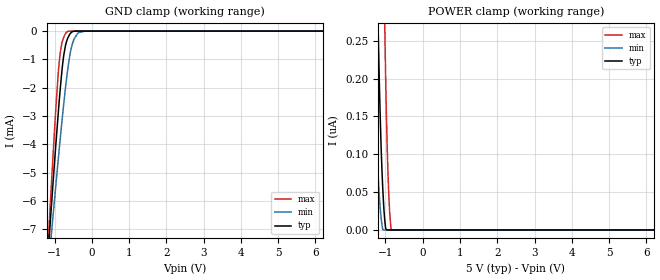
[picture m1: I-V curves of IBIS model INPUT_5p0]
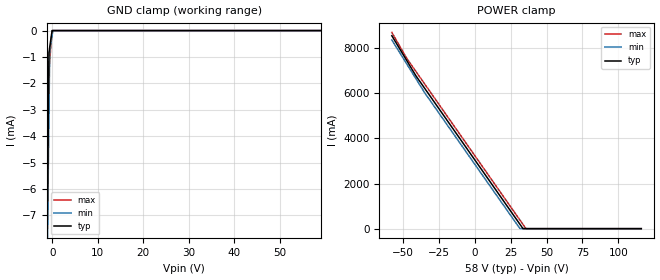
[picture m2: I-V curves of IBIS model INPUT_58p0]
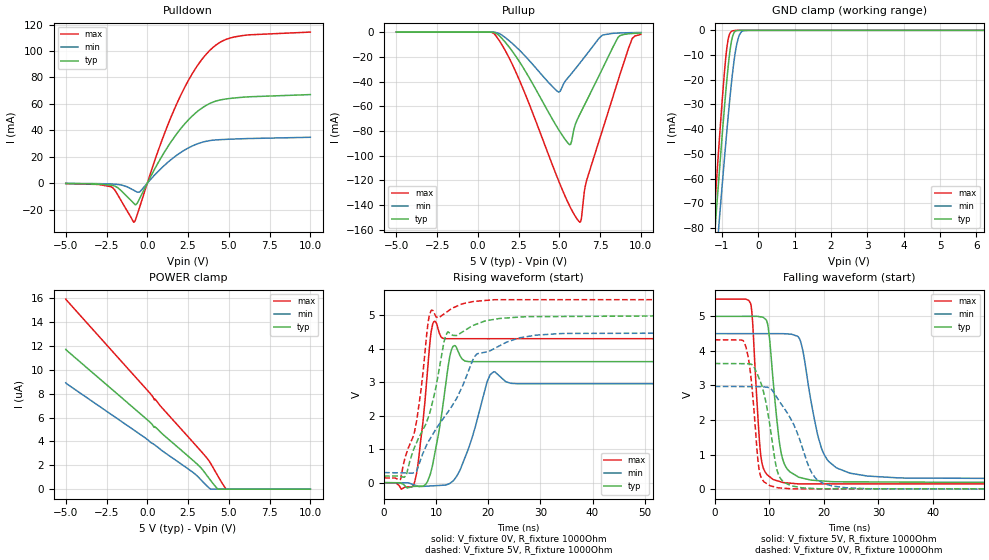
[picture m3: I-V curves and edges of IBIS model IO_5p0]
|Texas Instruments Incorporated
|TPS40170 4.5 V to 60 V, Wide-Input Synchronous PWM Buck Controller
[IBIS Ver]   4.1
[File name]   tps40170.ibs
[Date]   11/27/2018
[File Rev]   1.0
[Source]
| Texas Instruments Incorporated.
| Analog-eLab Design Center, HPA
| 12500 TI Blvd
| Dallas, TX -75243
[Notes]   Revision History:
| Rev 1.0: 11/27/2018
| - Initial version of the model
| - Model generated from simulations in SPECTRE
| - Warnings regarding combined Non-monotonicity of various models
|   have been reviewed and considered minor and can be ignored.
| - C_comp although listed in numerical order of value are
|   obtained from varying PVT conditions. For PVT conditions for
|   each specific value refer the buffer description under
|   respective [Model]. IBIS model user is responsible for using
|   appropriate C_comp to simulate for Signal Integrity.
| - Notes regarding non-monotonicity of various models
|   have been reviewed and considered minor and can be ignored.
| - Model names with a trailing _5 contain the model for 1.8V operation.
|   Model names with a trailing _58 contain the model for 3.3V operation.
|   Model names with a trailing _8 contain the model for 5.0V operation.
[Disclaimer]
| This model is designed as an aid for customers of Texas Instruments.
| TI and its licensors and suppliers make no warranties, either expressed
| or implied, with respect to this  model, including the warranties of
| merchantability or fitness for a particular purpose. The model is
| provided solely on an "as is" basis. The entire risk as to its quality
| and performance is with the customer.
| This model is subject to change without notice. Texas Instruments
| Incorporated is not responsible for updating this model.
[Copyright]
(C) Copyright 2018 Texas Instruments Incorporated.All rights reserved.
|  Component TPS40170RGY 20-pin VQFN - RGY package
|  Part # TPS40170RGY
[Component]   TPS40170RGY
[Manufacturer]  TI
[Package]   |20 VQFN - RGY package
|   typ   min   max
R_pkg   0.05   0.04   0.06
L_pkg   1.0nH   0.8nH   1.2nH
C_pkg   0.2pF   0.16pF   0.24pF
[Pin] signal_name   model_name   R_pin   L_pin   C_pin
1   ENABLE   INPUT   NA   NA   NA
2   SYNC   IO   NA   NA   NA
3   M/S   NC   NA   NA   NA
4   RT   NC   NA   NA   NA
5   SS   NC   NA   NA   NA
6   TRK   NC   NA   NA   NA
7   FB   NC   NA   NA   NA
8   COMP   NC   NA   NA   NA
9   AGND   GND   NA   NA   NA
10   VDD   POWER   NA   NA   NA
11   PGOOD   NC   NA   NA   NA
12   ILIM   NC   NA   NA   NA
13   PGND   GND   NA   NA   NA
14   LDRV   NC   NA   NA   NA
15   VBP   NC   NA   NA   NA
16   SW   NC   NA   NA   NA
17   HDRV   NC   NA   NA   NA
18   BOOT   NC   NA   NA   NA
19   VIN   POWER   NA   NA   NA
20   UVLO   NC   NA   NA   NA
[Model Selector] INPUT
INPUT_5p0   5.0V   digital Input
INPUT_58p0   58.0V  digital Input
[Model Selector] IO
IO_5p0   5.0V  digital I/O
IO_8p0   8.0V  digital I/O
| Models and submodels in the file (4): INPUT_5p0 (Input), INPUT_58p0 (Input), IO_5p0 (I/O), IO_8p0 (I/O)
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|   INPUT_5p0 Model
[Model]   INPUT_5p0
Model_type   Input
Vinl = 0.1
Vinh = 0.6
|   typ   min   max
C_comp   4.463E-13   4.443E-13   4.804E-13
|  Where Nom  PVT is Nominal Process, 5.0V,  27C
|   Fast PVT is Strong Process,  5.5V, -40C
|   Slow PVT is Weak Process,   4.5V, 125C
[Voltage Range]   5   4.5   5.5
|Junction Temperature
[Temperature Range]   27   125   -40
[Power Clamp Reference]   5   4.5   5.5
[GND Clamp Reference]   0   0   0
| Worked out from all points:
|   GND clamp passes 1 mA (typ) near -0.77 V on its own axis
[GND Clamp]
|   Voltage   I(typ)   I(min)   I(max)
-5V       -86.97mA   -70.6mA    -108.1mA
-1.25V    -9.29mA    -9.605mA   -9.357mA
-1.13V    -6.99mA    -7.811mA   -6.43mA
-1.07V    -5.864mA   -6.927mA   -5.009mA
-965mV    -3.955mA   -5.407mA   -2.669mA
-860mV    -2.197mA   -3.939mA   -875.2uA
-755mV    -847.5uA   -2.559mA   -211.6uA
-650mV    -253.7uA   -1.36mA    -12.81uA
-560mV    -56.52uA   -634.1uA   -388.1nA
-470mV    -3.429uA   -258.8uA   -54.84nA
-170mV    -39.22nA   -485.2nA   -50.33nA
10V       0A         0A         0A
[POWER Clamp]
|   Voltage   I(typ)   I(min)   I(max)
-5V       66.16uA    47.89uA    96.51uA
-1.655V   2.175uA    1.129uA    4.477uA
-1.25V    408.6nA    131nA      1.384uA
-1.205V   286.4nA    79.41nA    1.113uA
-1.19V    250.8nA    65.2nA     1.029uA
-1.115V   107.4nA    15.29nA    642.3nA
-1.07V    52.12nA    72.28pA    448.7nA
-1.025V   16.43nA    0A         288.1nA
-935mV    0A         0A         79.11nA
-890mV    0A         0A         25.91nA
-845mV    0A         0A         276.1pA
10V       0A         0A         0A
|   INPUT_58p0 Model
[Model]   INPUT_58p0
Model_type   Input
Vinl = 0.1
Vinh = 0.6
|   typ   min   max
C_comp   4.760E-13   3.805E-13   4.871E-13
|  Where Nom  PVT is Nominal Process, 58V,  27C
|   Fast PVT is Strong Process,  60V, -40C
|   Slow PVT is Weak Process,   56V, 125C
[Voltage Range]   58   56   60
|Junction Temperature
[Temperature Range]   27   125   -40
[Power Clamp Reference]   58   56   60
[GND Clamp Reference]   0   0   0
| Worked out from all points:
|   GND clamp passes 1 mA (typ) near -0.76 V on its own axis
[GND Clamp]
|   Voltage   I(typ)   I(min)   I(max)
-58V      -5.49A     -5.046A    -5.928A
-2.146V   -27.23mA   -23.55mA   -32.3mA
-928mV    -4.137mA   -5.827mA   -1.934mA
-754mV    -838.2uA   -3.295mA   -1.547mA
-580mV    -628.6uA   -762.6uA   -1.16mA
-58mV     -20.47fA   -190.7uA   -51.12fA
116mV     0A         0A         0A
116V      0A         0A         0A
[POWER Clamp]
|   Voltage   I(typ)   I(min)   I(max)
-58V      8.556A     8.365A     8.702A
-47.39V   7.432A     7.282A     7.532A
-40.95V   6.754A     6.626A     6.947A
-34.68V   6.186A     5.99A      6.378A
31.44V    186.8mA    6.365mA    373.9mA
33.52V    5.407mA    346.3uA    185.3mA
35.79V    335uA      268.4uA    503.6uA
116V      0A         0A         0A
|   IO_5p0 Model
[Model]   IO_5p0
Model_type   I/O
Polarity   Non-Inverting
Enable   Active-High
Vinl = 0.8
Vinh = 2
Vmeas = 2.5
Vref = 0
Cref = 2pF
Rref = 100000
|   typ   min   max
C_comp   2.387E-12   1.948E-12   2.498E-12
|  Where Nom  PVT is Nominal Process, 5.0V,  27C
|   Fast PVT is Strong Process,  5.5V, -40C
|   Slow PVT is Weak Process,   4.5V, 125C
[Voltage Range]   5   4.5   5.5
|Junction Temperature
[Temperature Range]   27   125   -40
[Pullup Reference]   5   4.5   5.5
[Pulldown Reference]   -0   0   0
[Power Clamp Reference]   5   4.5   5.5
[GND Clamp Reference]   0   0   0
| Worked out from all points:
|   slope of the pulldown table from 0 to 0.75 V, typ, clamps not added: 43.5 ohm
|   slope of the pullup table from 0 to 0.75 V, typ, clamps not added: 36 kohm
|   GND clamp passes 1 mA (typ) near -0.67 V on its own axis
|   falling waveform, V_fixture 5V, R_fixture 1000Ohm: 20-80 % time 1.82ns typ, 3.13ns min, 1.2ns max; typ from 4.99 V to 0.198 V
|   rising waveform, V_fixture 0V, R_fixture 1000Ohm: 20-80 % time 2.25ns typ, 3.56ns min, 1.65ns max; typ from 0 V to 3.63 V
|   rising waveform, V_fixture 5V, R_fixture 1000Ohm: 20-80 % time 5.18ns typ, 8.8ns min, 3.05ns max; typ from 0.198 V to 4.99 V
|   falling waveform, V_fixture 0V, R_fixture 1000Ohm: 20-80 % time 2.38ns typ, 4.83ns min, 1.43ns max; typ from 3.63 V to 0 V
[Pulldown]
|   Voltage   I(typ)   I(min)   I(max)
-5V       -233.1uA   -135.6uA   -319.7uA
-2.165V   -1.626mA   -658.4uA   -3.098mA
-800mV    -15.63mA   -5.555mA   -29.46mA
-620mV    -15.28mA   -6.757mA   -23.97mA
-455mV    -11.28mA   -6.464mA   -17.64mA
640mV     14.89mA    8.596mA    23.64mA
1.69V     35.41mA    20.08mA    56.84mA
2.74V     50.64mA    28.03mA    82.5mA
3.79V     60.07mA    32.14mA    99.97mA
4.495V    63.05mA    32.96mA    106.9mA
5.47V     64.65mA    33.48mA    111mA
10V       67.05mA    34.74mA    114.4mA
[GND Clamp]
|   Voltage   I(typ)   I(min)   I(max)
-5V       -893.1mA   -848.5mA   -967.2mA
-1.25V    -92.33mA   -109.2mA   -82.83mA
-1.13V    -68.55mA   -87.15mA   -56.65mA
-1.07V    -56.91mA   -76.29mA   -43.93mA
-935mV    -31.84mA   -52.49mA   -17.5mA
-875mV    -21.64mA   -42.35mA   -8.248mA
-800mV    -10.7mA    -30.31mA   -1.899mA
-710mV    -2.577mA   -17.45mA   -244.9uA
-590mV    -85.03uA   -5.428mA   -18.61uA
-515mV    -7.368uA   -1.701mA   -2.317uA
-410mV    -77.06nA   -152uA     0A
10V       0A         0A         0A
[Pullup]
|   Voltage   I(typ)   I(min)   I(max)
-5V       1.348nA    7.768nA    176.2pA
1.045V    -456uA     -166uA     -1.981mA
2.53V     -23.56mA   -14.36mA   -38.38mA
4.945V    -78.74mA   -48.48mA   -120.1mA
5.62V     -91.05mA   -35.45mA   -140.4mA
6.265V    -66.18mA   -24.91mA   -153.8mA
6.355V    -63.81mA   -23.4mA    -150.2mA
6.67V     -55.55mA   -18.07mA   -119.9mA
7.645V    -29.48mA   -2.42mA    -79.13mA
8.59V     -4.385mA   -777.5uA   -39.42mA
9.46V     -1.137mA   -458uA     -5.377mA
10V       -784.7uA   -349.9uA   -1.864mA
[POWER Clamp]
|   Voltage   I(typ)   I(min)   I(max)
-5V       11.72uA    8.915uA    15.93uA
-185mV    6.032uA    4.352uA    8.573uA
220mV     5.539uA    3.905uA    7.953uA
430mV     5.208uA    3.73uA     7.481uA
475mV     5.224uA    3.686uA    7.544uA
880mV     4.687uA    3.254uA    6.854uA
3.01V     2.157uA    1.171uA    3.618uA
3.37V     1.662uA    671.9nA    3.063uA
3.88V     738.9nA    3.334nA    2.171uA
4.33V     534.8pA    0A         1.103uA
4.84V     0A         0A         174.1pA
10V       0A         0A         0A
[Ramp]
R_load = 1000
|   typ   min   max
dV/dt_r   2.17919/2.23232e-09   1.78064/3.51242e-09   2.59027/1.64795e-09
dV/dt_f   2.87733/1.81661e-09   2.51629/3.13168e-09   3.21128/1.20016e-09
[Falling Waveform]
V_fixture = 5V
V_fixture_min = 4.5V
V_fixture_max = 5.5V
R_fixture = 1000Ohm
C_fixture = 0F
|   Time   V(typ)   V(min)   V(max)
0s        4.994V     4.496V     5.492V
6.601ns   4.995V     4.495V     5.35V
8.311ns   4.983V     4.495V     1.183V
9.478ns   4.882V     4.495V     441.5mV
12.18ns   1.043V     4.494V     208.3mV
15.26ns   358.8mV    4.406V     153.4mV
18.82ns   248mV      1.6V       153.4mV
20.57ns   226.7mV    864mV      153.3mV
33.55ns   205.4mV    327.1mV    153.1mV
833.4ns   198.5mV    301.8mV    139.5mV
[Rising Waveform]
V_fixture = 0V
V_fixture_min = 0V
V_fixture_max = 0V
R_fixture = 1000Ohm
C_fixture = 0F
|   Time   V(typ)   V(min)   V(max)
0s        -445nV     4.035uV    -316.9nV
5.871ns   -110.5mV   -72.44mV   24.46mV
7.408ns   -103.6mV   -112.1mV   1.75V
8.963ns   311.2mV    -98.03mV   4.434V
9.681ns   836.4mV    -91.53mV   4.827V
13.12ns   4.048V     37.13mV    4.305V
16.06ns   3.623V     967mV      4.305V
21.03ns   3.619V     3.316V     4.305V
25.53ns   3.619V     2.96V      4.305V
833.4ns   3.632V     2.968V     4.317V
[Rising Waveform]
V_fixture = 5V
V_fixture_min = 4.5V
V_fixture_max = 5.5V
R_fixture = 1000Ohm
C_fixture = 0F
|   Time   V(typ)   V(min)   V(max)
0s        198.5mV    301.8mV    139.5mV
3.11ns    188.1mV    292.7mV    94.64mV
4.245ns   212.6mV    289.3mV    857.6mV
5.775ns   1.035V     305.9mV    1.487V
8.963ns   2.205V     1.348V     5.132V
12.11ns   4.488V     2.083V     5.114V
17.35ns   4.719V     3.766V     5.423V
21.16ns   4.885V     4.012V     5.472V
34.93ns   4.971V     4.464V     5.472V
833.4ns   4.994V     4.496V     5.492V
[Falling Waveform]
|Gnd
V_fixture = 0V
V_fixture_min = 0V
V_fixture_max = 0V
R_fixture = 1000Ohm
C_fixture = 0F
|   Time   V(typ)   V(min)   V(max)
0s        3.632V     2.968V     4.317V
5.439ns   3.626V     2.965V     4.242V
7.173ns   3.543V     2.964V     2.323V
7.964ns   3.27V      2.963V     770.7mV
8.552ns   3.031V     2.959V     326.4mV
11.45ns   536.9mV    2.637V     45.44mV
14.05ns   97.15mV    2V         9.64mV
18.82ns   13.54mV    268.6mV    9.584mV
28.47ns   10.16mV    11.72mV    9.47mV
833.4ns   -594.7nV   3.765uV    -316.8nV
